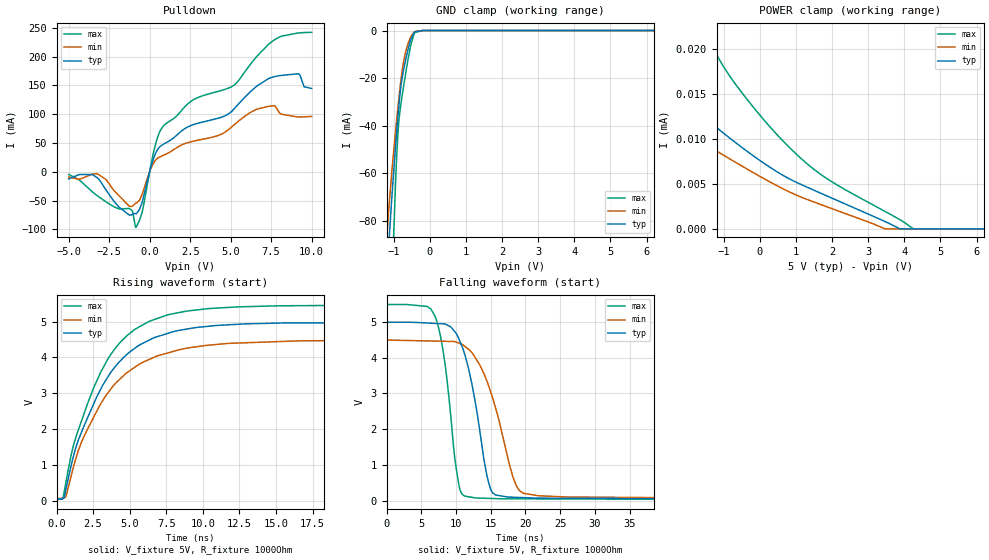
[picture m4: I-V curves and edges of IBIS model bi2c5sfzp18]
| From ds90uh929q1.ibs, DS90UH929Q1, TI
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|   Model
[Model]   bi2c5sfzp18
Model_type   I/O_open_drain
Polarity   Non-Inverting
Enable   Active-Low
Vinl = 1.5
Vinh = 3.5
Vmeas = 2.5
Vref = 5
Cref = 1pF
Rref = 1000
|   typ   min   max
C_comp   0.116pF   0.078pF   0.210pF
[Voltage Range]   5   4.5   5.5
[Temperature Range]   27   105   -40
[Pullup Reference]   5   4.5   5.5
[Pulldown Reference]   0   0   0
[Power Clamp Reference]   5   4.5   5.5
[GND Clamp Reference]   0   0   0
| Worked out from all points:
|   slope of the pulldown table from 0 to 0.75 V, typ, clamps not added: 16.3 ohm
|   GND clamp passes 1 mA (typ) near -0.44 V on its own axis
|   POWER clamp passes 1 mA (typ) near -4.25 V on its own axis
|   falling waveform, V_fixture 5V, R_fixture 1000Ohm: 20-80 % time 2.74ns typ, 3.89ns min, 1.91ns max; typ from 4.99 V to 0.049 V
|   rising waveform, V_fixture 5V, R_fixture 1000Ohm: 20-80 % time 3.55ns typ, 3.75ns min, 3.36ns max; typ from 0.046 V to 4.99 V
[Pulldown]
|   Voltage   I(typ)   I(min)   I(max)
-5V       -12.46mA   -9.13mA    -4.715mA
-3.53V    -4.967mA   -4.024mA   -35.17mA
-1.085V   -74.7mA    -60.21mA   -67.46mA
-830mV    -73.22mA   -54.4mA    -96.25mA
-455mV    -52.16mA   -38.52mA   -69.26mA
310mV     28.17mA    18.1mA     41.76mA
835mV     47.62mA    28.33mA    79.23mA
2.71V     81.92mA    53.09mA    125.2mA
5.26V     110.6mA    82.57mA    151.3mA
7.465V    163.2mA    114.1mA    224.2mA
9.19V     170.1mA    95.09mA    241mA
10V       144.6mA    96mA       242.1mA
[GND Clamp]
|   Voltage   I(typ)   I(min)   I(max)
-5V       -1.642A    -1.67A     -2.408A
-1.25V    -121mA     -99.88mA   -207.3mA
-1.16V    -95.91mA   -79.77mA   -161mA
-1.13V    -88.29mA   -73.73mA   -146mA
-1.01V    -61.06mA   -52.1mA    -89.38mA
-905mV    -39.98mA   -35.47mA   -48.82mA
-830mV    -27.22mA   -24.58mA   -34.19mA
-755mV    -18.82mA   -15.62mA   -26.19mA
-665mV    -11.95mA   -8.707mA   -17.55mA
-515mV    -3.227mA   -2.241mA   -5.347mA
-410mV    -504.7uA   -404.8uA   -785.2uA
10V       0A         0A         0A
[POWER Clamp]
|   Voltage   I(typ)   I(min)   I(max)
-5V       106.1mA    281mA      3.954mA
-3.845V   22.26uA    68.81mA    804uA
-3.2V     18.92uA    92.19uA    273.4uA
-1.25V    11.45uA    8.794uA    19.81uA
-830mV    10.09uA    7.784uA    16.97uA
-275mV    8.404uA    6.48uA     14.01uA
1.06V     5.094uA    3.679uA    8.133uA
1.9V      3.598uA    2.4uA      5.481uA
3.46V     838.6nA    21.7nA     1.963uA
3.865V    25.11nA    0A         1.066uA
4.24V     0A         0A         35.63nA
10V       0A         0A         0A
[Ramp]
R_load = 1000
|   typ   min   max
dV/dt_r   2.96444/3.54778e-09   2.65697/3.73177e-09   3.26664/3.36293e-09
dV/dt_f   2.96582/2.72588e-09   2.65372/3.86852e-09   3.27017/1.89823e-09
[Falling Waveform]
V_fixture = 5V
V_fixture_min = 4.5V
V_fixture_max = 5.5V
R_fixture = 1000Ohm
C_fixture = 0F
|   Time   V(typ)   V(min)   V(max)
0s        4.992V     4.493V     5.487V
6.93ns    4.959V     4.464V     5.183V
8.445ns   4.942V     4.457V     3.796V
10.32ns   4.572V     4.415V     553.2mV
11.15ns   4.159V     4.335V     138.5mV
14.44ns   729.1mV    3.355V     65.14mV
15.62ns   169.1mV    2.652V     57.73mV
18.18ns   95.35mV    681.1mV    50.47mV
19.75ns   84.13mV    207.8mV    49.8mV
50ns      49mV       70.59mV    36.85mV
[Rising Waveform]
V_fixture = 5V
V_fixture_min = 4.5V
V_fixture_max = 5.5V
R_fixture = 1000Ohm
C_fixture = 0F
|   Time   V(typ)   V(min)   V(max)
0s        46.22mV    61.2mV     35.9mV
443.4ps   61.01mV    65.08mV    65.64mV
636.8ps   298.2mV    107.5mV    502.1mV
1.132ns   1.198V     900mV      1.51V
1.489ns   1.689V     1.399V     1.972V
3.489ns   3.442V     2.999V     3.943V
5.285ns   4.237V     3.709V     4.764V
7.576ns   4.67V      4.123V     5.187V
16.63ns   4.965V     4.465V     5.448V
50ns      4.987V     4.489V     5.48V
